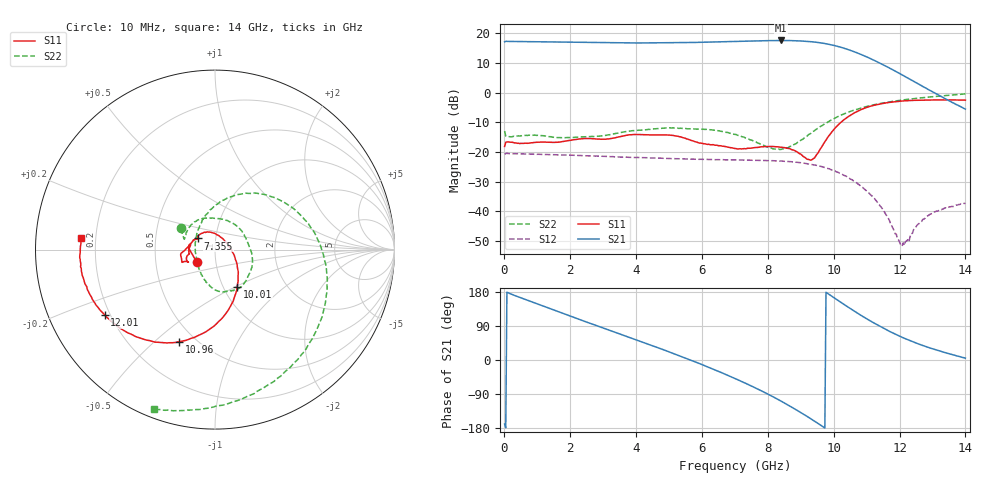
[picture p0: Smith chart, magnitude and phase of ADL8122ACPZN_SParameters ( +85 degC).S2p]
! "Analog Devices, Inc."
! Device:	ADL8122ACPZN
! Description:	"10 kHz to 10 GHz, Wideband, Low Noise Amplifier"
! Conditions:	Vdd = 5.0 V
!		IDQ = 95 mA
!		Pin = -25 dBm
!		Operating Temperature = +25 C (at package bottom)
! Product validation unit SN1 soldered down to Evaluation Board as shown on ADL8122-EVALZ User Guide. Board loss de-embedded from S21 magnitude.  All other RF measurements reference to RF coaxial connector.
! Frequency (GHz)	S11_Mag (dB)	S11_Phase (deg)	S21_Mag (dB)	S21_Phase (deg)	S12_Mag (dB)	S12_Phase (deg)	S22_Mag (dB)	S22_Phase (deg)
#  GHZ  S  DB  R 50
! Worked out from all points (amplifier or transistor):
!   401 points, 10 MHz to 14 GHz, reference 50 ohm
!   highest |S21| = 17.6 dB at 8.404 GHz (marker M1)
!   |S21| within 3 dB of that: start of sweep to 10.42 GHz
!   unconditionally stable (mu >= 1): start of sweep to end of sweep
!   at 2.318 GHz: K = 1.11, MAG = 17.1 dB, |S12| = -21.2 dB
!   at 7.005 GHz: K = 1.15, MAG = 17.6 dB, |S12| = -22.7 dB
!   at 14 GHz: K = 2.55, MAG = 9.0 dB, |S12| = -37.4 dB
!   S11 on the Smith chart (normalised r, x): 10 MHz: 0.81, -0.11; 7.355 GHz: 0.82, +0.10; 10.01 GHz: 1.16, -0.51; 10.96 GHz: 0.41, -0.60; 12.01 GHz: 0.18, -0.26; 14 GHz: 0.14, +0.04
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0.01  -18.18 -145.8  17.13 -168.9  -20.78 10.0  -12.97 148.4
0.21985  -16.73 169.2  17.27 173.5  -20.60 -5.0  -14.93 157.0
1.094225  -16.71 -177.6  17.15 144.9  -20.84 -27.4  -14.47 117.9
2.353325  -15.58 -162.8  16.93 104.6  -21.24 -59.0  -14.95 46.9
3.472525  -14.96 -158.2  16.76 69.9  -21.68 -87.4  -13.60 -9.3
4.69665  -14.28 -168.8  16.77 31.4  -22.09 -120.7  -12.09 -49.6
5.920775  -17.02 169.0  16.96 -9.2  -22.50 -155.9  -12.36 -75.0
6.4454  -17.73 154.9  17.09 -27.9  -22.62 -171.5  -12.78 -87.0
7.005  -18.86 148.8  17.25 -48.9  -22.71 171.1  -14.09 -101.4
7.35475  -18.89 146.8  17.36 -62.6  -22.75 159.5  -15.36 -113.1
7.91435  -18.17 147.3  17.51 -86.1  -22.90 140.7  -18.04 -140.1
8.404  -18.43 135.4  17.59 -108.5  -23.10 122.6  -19.16 177.9
8.858675  -19.79 107.7  17.48 -131.2  -23.48 104.3  -17.23 134.0
9.348325  -22.56 30.4  17.14 -157.4  -24.28 83.0  -13.34 98.8
9.6631  -17.82 -26.8  16.69 -175.3  -25.02 68.3  -11.05 80.0
10.01285  -12.39 -59.0  15.91 164.3  -26.33 50.8  -8.77 59.3
10.46752  -7.94 -87.0  14.42 137.9  -28.81 28.6  -6.52 32.8
10.95717  -5.18 -111.3  12.27 111.1  -32.77 4.0  -4.81 5.7
11.69165  -3.29 -139.9  8.32 75.8  -43.04 -41.1  -3.11 -30.7
12.00642  -2.92 -149.5  6.42 62.8  -50.55 -86.6  -2.62 -44.7
12.8808  -2.49 -168.1  0.97 33.2  -41.41 147.6  -1.51 -78.3
14  -2.53 175.0  -5.57 4.8  -37.43 121.0  -0.42 -110.9
